(* Logix 5000 AddOnInstructionDefinition export Banner_TL70Pro_Param_v4; software revision 33.00; part 3 of 3 *)
(* tags used below, declared in another part *)
   TL70Pro : Banner_TL70Pro_v4;
   Port_Data : Banner_IOL_Port_v4;
   Port : INT;   // Port Number that device is plugged into.
   Local_Control : DINT;
   Command_Being_Processed : BOOL;
   Update_Archive : BOOL;
   Index_Write_Inprocess : DINT;
   Inprocess_Index : DINT;
   W_Index : DINT;
(* Banner_TL70Pro_Param_v4, continued *)

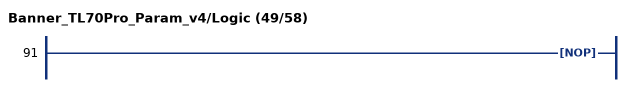
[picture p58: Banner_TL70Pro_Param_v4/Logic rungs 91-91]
   91: NOP();
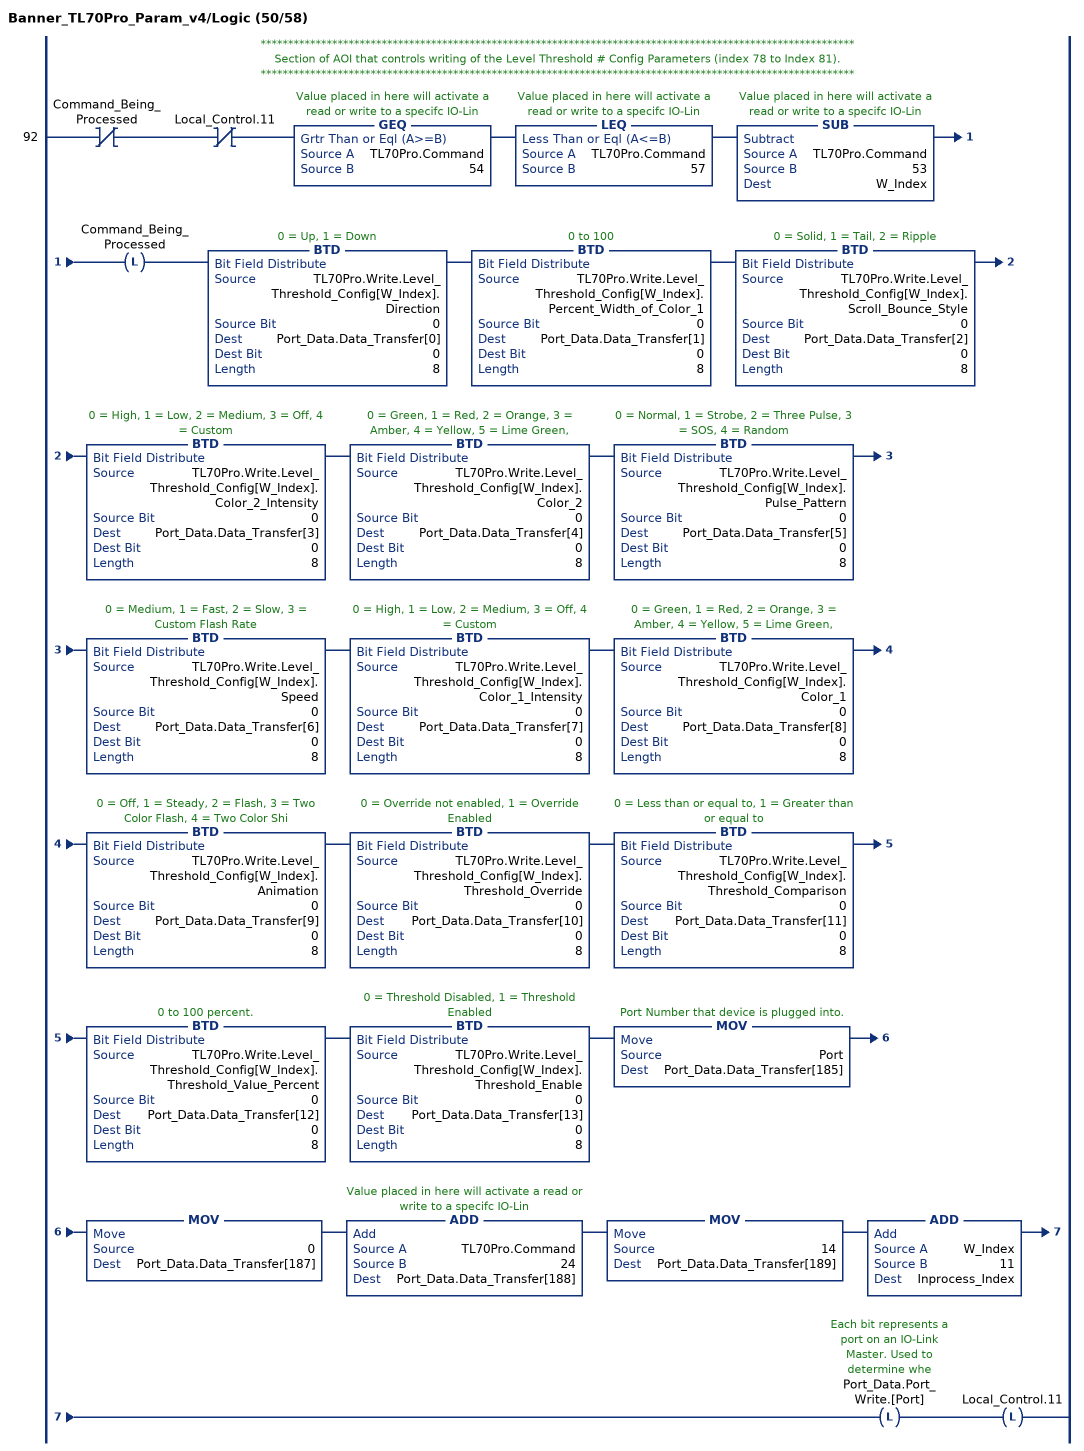
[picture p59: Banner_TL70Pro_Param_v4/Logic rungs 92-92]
   // ************************************************************************************************************
   // Section of AOI that controls writing of the Level Threshold # Config Parameters (index 78 to Index 81).
   // ************************************************************************************************************
   92: XIO(Command_Being_Processed)XIO(Local_Control.11)GEQ(TL70Pro.Command,54)LEQ(TL70Pro.Command,57)SUB(TL70Pro.Command,53,W_Index)OTL(Command_Being_Processed)BTD(TL70Pro.Write.Level_Threshold_Config[W_Index].Direction,0,Port_Data.Data_Transfer[0],0,8)BTD(TL70Pro.Write.Level_Threshold_Config[W_Index].Percent_Width_of_Color_1,0,Port_Data.Data_Transfer[1],0,8)BTD(TL70Pro.Write.Level_Threshold_Config[W_Index].Scroll_Bounce_Style,0,Port_Data.Data_Transfer[2],0,8)BTD(TL70Pro.Write.Level_Threshold_Config[W_Index].Color_2_Intensity,0,Port_Data.Data_Transfer[3],0,8)BTD(TL70Pro.Write.Level_Threshold_Config[W_Index].Color_2,0,Port_Data.Data_Transfer[4],0,8)BTD(TL70Pro.Write.Level_Threshold_Config[W_Index].Pulse_Pattern,0,Port_Data.Data_Transfer[5],0,8)BTD(TL70Pro.Write.Level_Threshold_Config[W_Index].Speed,0,Port_Data.Data_Transfer[6],0,8)BTD(TL70Pro.Write.Level_Threshold_Config[W_Index].Color_1_Intensity,0,Port_Data.Data_Transfer[7],0,8)BTD(TL70Pro.Write.Level_Threshold_Config[W_Index].Color_1,0,Port_Data.Data_Transfer[8],0,8)BTD(TL70Pro.Write.Level_Threshold_Config[W_Index].Animation,0,Port_Data.Data_Transfer[9],0,8)BTD(TL70Pro.Write.Level_Threshold_Config[W_Index].Threshold_Override,0,Port_Data.Data_Transfer[10],0,8)BTD(TL70Pro.Write.Level_Threshold_Config[W_Index].Threshold_Comparison,0,Port_Data.Data_Transfer[11],0,8)BTD(TL70Pro.Write.Level_Threshold_Config[W_Index].Threshold_Value_Percent,0,Port_Data.Data_Transfer[12],0,8)BTD(TL70Pro.Write.Level_Threshold_Config[W_Index].Threshold_Enable,0,Port_Data.Data_Transfer[13],0,8)MOV(Port,Port_Data.Data_Transfer[185])MOV(0,Port_Data.Data_Transfer[187])ADD(TL70Pro.Command,24,Port_Data.Data_Transfer[188])MOV(14,Port_Data.Data_Transfer[189])ADD(W_Index,11,Inprocess_Index)OTL(Port_Data.Port_Write.[Port])OTL(Local_Control.11);
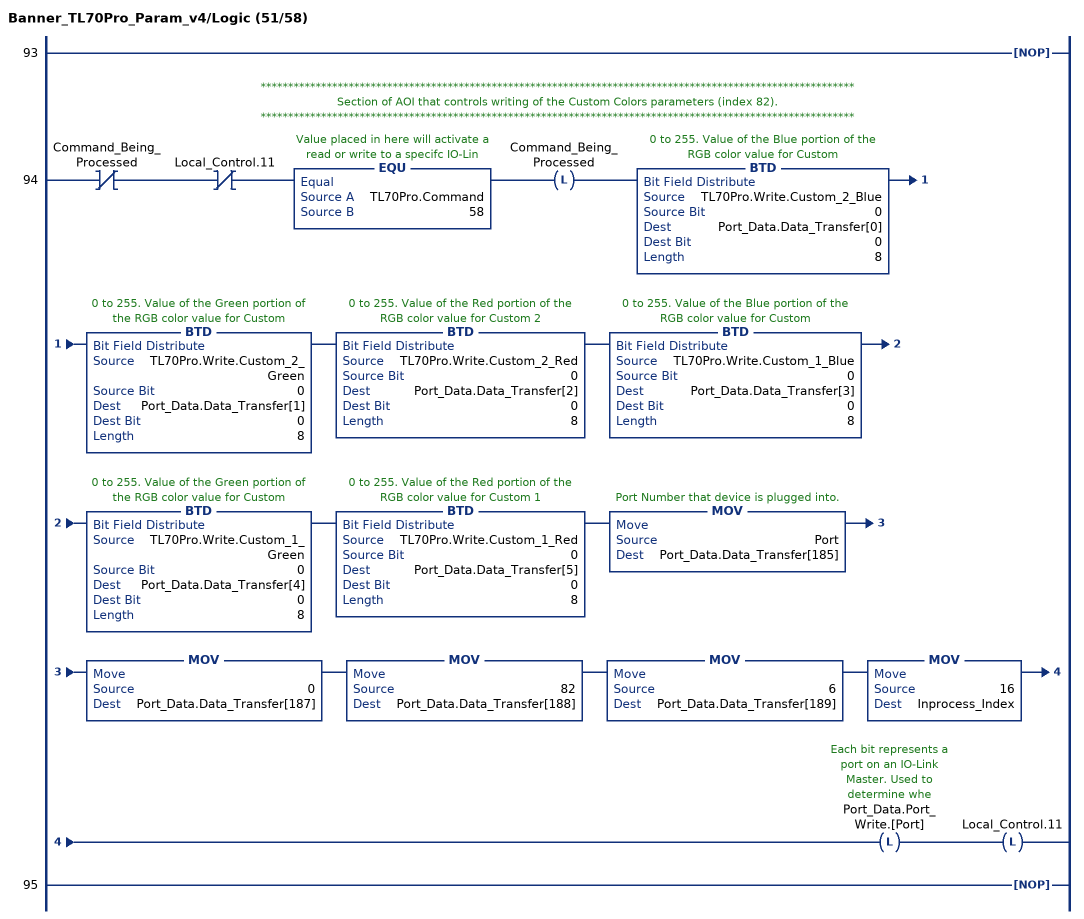
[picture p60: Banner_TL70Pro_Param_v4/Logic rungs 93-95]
   93: NOP();
   // ************************************************************************************************************
   // Section of AOI that controls writing of the Custom Colors parameters (index 82).
   // ************************************************************************************************************
   94: XIO(Command_Being_Processed)XIO(Local_Control.11)EQU(TL70Pro.Command,58)OTL(Command_Being_Processed)BTD(TL70Pro.Write.Custom_2_Blue,0,Port_Data.Data_Transfer[0],0,8)BTD(TL70Pro.Write.Custom_2_Green,0,Port_Data.Data_Transfer[1],0,8)BTD(TL70Pro.Write.Custom_2_Red,0,Port_Data.Data_Transfer[2],0,8)BTD(TL70Pro.Write.Custom_1_Blue,0,Port_Data.Data_Transfer[3],0,8)BTD(TL70Pro.Write.Custom_1_Green,0,Port_Data.Data_Transfer[4],0,8)BTD(TL70Pro.Write.Custom_1_Red,0,Port_Data.Data_Transfer[5],0,8)MOV(Port,Port_Data.Data_Transfer[185])MOV(0,Port_Data.Data_Transfer[187])MOV(82,Port_Data.Data_Transfer[188])MOV(6,Port_Data.Data_Transfer[189])MOV(16,Inprocess_Index)OTL(Port_Data.Port_Write.[Port])OTL(Local_Control.11);
   95: NOP();
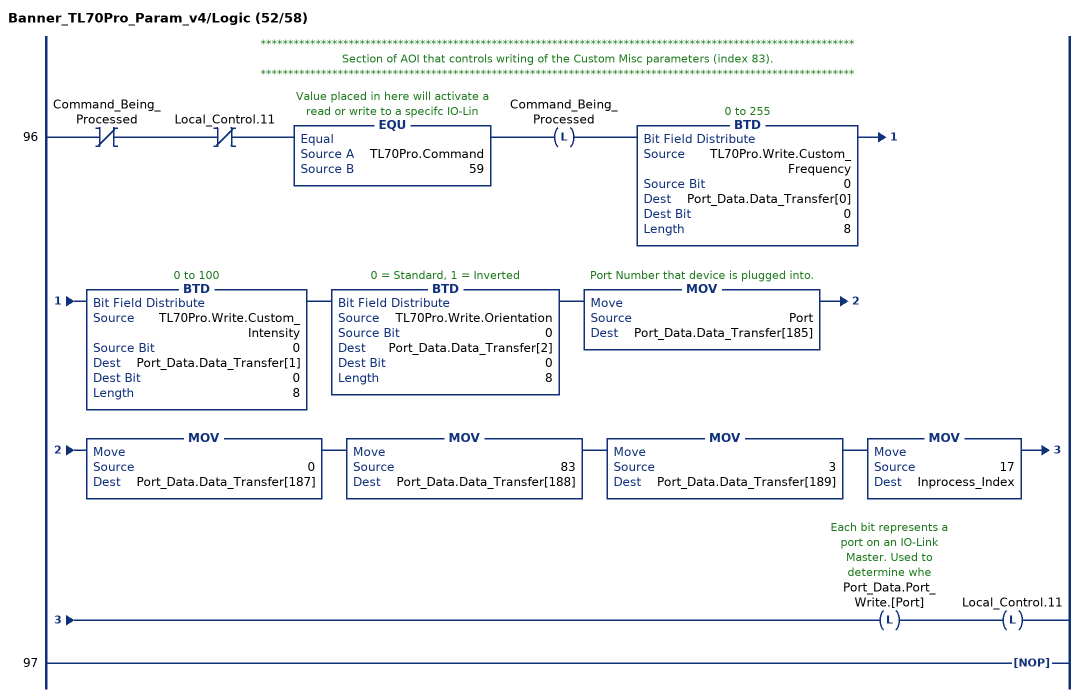
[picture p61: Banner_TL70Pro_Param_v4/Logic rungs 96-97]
   // ************************************************************************************************************
   // Section of AOI that controls writing of the Custom Misc parameters (index 83).
   // ************************************************************************************************************
   96: XIO(Command_Being_Processed)XIO(Local_Control.11)EQU(TL70Pro.Command,59)OTL(Command_Being_Processed)BTD(TL70Pro.Write.Custom_Frequency,0,Port_Data.Data_Transfer[0],0,8)BTD(TL70Pro.Write.Custom_Intensity,0,Port_Data.Data_Transfer[1],0,8)BTD(TL70Pro.Write.Orientation,0,Port_Data.Data_Transfer[2],0,8)MOV(Port,Port_Data.Data_Transfer[185])MOV(0,Port_Data.Data_Transfer[187])MOV(83,Port_Data.Data_Transfer[188])MOV(3,Port_Data.Data_Transfer[189])MOV(17,Inprocess_Index)OTL(Port_Data.Port_Write.[Port])OTL(Local_Control.11);
   97: NOP();
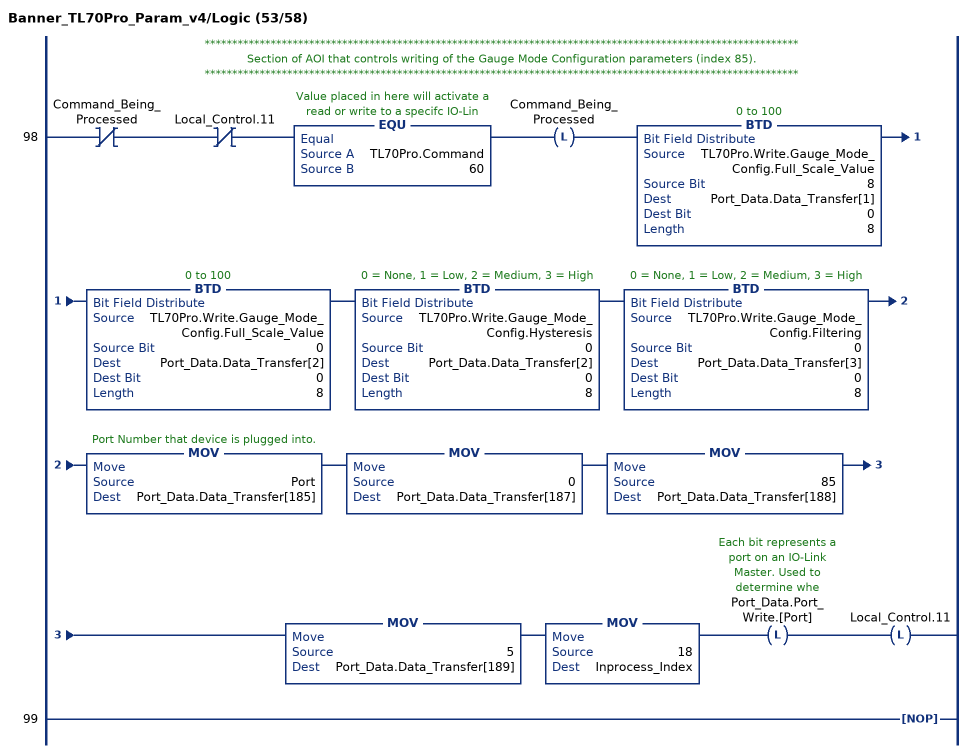
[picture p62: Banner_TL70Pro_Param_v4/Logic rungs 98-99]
   // ************************************************************************************************************
   // Section of AOI that controls writing of the Gauge Mode Configuration parameters (index 85).
   // ************************************************************************************************************
   98: XIO(Command_Being_Processed)XIO(Local_Control.11)EQU(TL70Pro.Command,60)OTL(Command_Being_Processed)BTD(TL70Pro.Write.Gauge_Mode_Config.Full_Scale_Value,8,Port_Data.Data_Transfer[1],0,8)BTD(TL70Pro.Write.Gauge_Mode_Config.Full_Scale_Value,0,Port_Data.Data_Transfer[2],0,8)BTD(TL70Pro.Write.Gauge_Mode_Config.Hysteresis,0,Port_Data.Data_Transfer[2],0,8)BTD(TL70Pro.Write.Gauge_Mode_Config.Filtering,0,Port_Data.Data_Transfer[3],0,8)MOV(Port,Port_Data.Data_Transfer[185])MOV(0,Port_Data.Data_Transfer[187])MOV(85,Port_Data.Data_Transfer[188])MOV(5,Port_Data.Data_Transfer[189])MOV(18,Inprocess_Index)OTL(Port_Data.Port_Write.[Port])OTL(Local_Control.11);
   99: NOP();
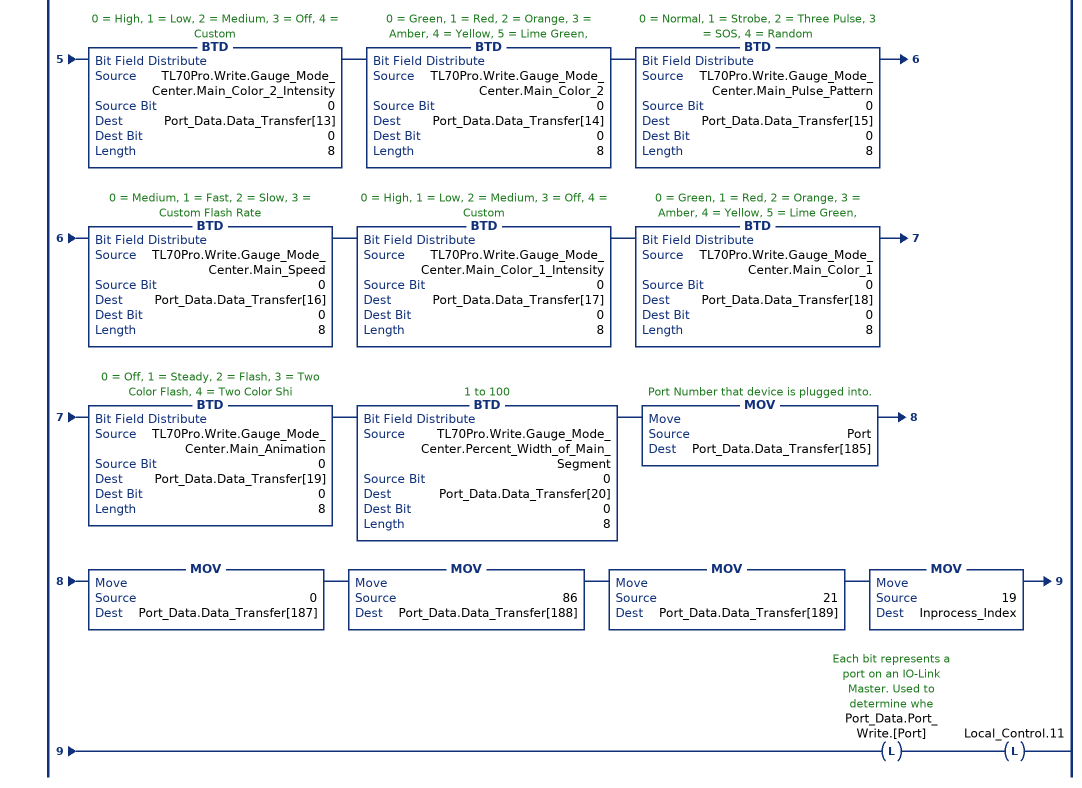
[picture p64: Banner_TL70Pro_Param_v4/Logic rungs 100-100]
   // ************************************************************************************************************
   // Section of AOI that controls writing of the Gauge Mode Center Settings parameters (index 86).
   // ************************************************************************************************************
   100: XIO(Command_Being_Processed)XIO(Local_Control.11)EQU(TL70Pro.Command,61)OTL(Command_Being_Processed)BTD(TL70Pro.Write.Gauge_Mode_Center.BG_Direction,0,Port_Data.Data_Transfer[0],0,8)BTD(TL70Pro.Write.Gauge_Mode_Center.BG_Percent_Width_of_Color_1,0,Port_Data.Data_Transfer[1],0,8)BTD(TL70Pro.Write.Gauge_Mode_Center.BG_Scroll_Bounce_Style,0,Port_Data.Data_Transfer[2],0,8)BTD(TL70Pro.Write.Gauge_Mode_Center.BG_Color_2_Intensity,0,Port_Data.Data_Transfer[3],0,8)BTD(TL70Pro.Write.Gauge_Mode_Center.BG_Color_2,0,Port_Data.Data_Transfer[4],0,8)BTD(TL70Pro.Write.Gauge_Mode_Center.BG_Pulse_Pattern,0,Port_Data.Data_Transfer[5],0,8)BTD(TL70Pro.Write.Gauge_Mode_Center.BG_Speed,0,Port_Data.Data_Transfer[6],0,8)BTD(TL70Pro.Write.Gauge_Mode_Center.BG_Color_1_Intensity,0,Port_Data.Data_Transfer[7],0,8)BTD(TL70Pro.Write.Gauge_Mode_Center.BG_Color_1,0,Port_Data.Data_Transfer[8],0,8)BTD(TL70Pro.Write.Gauge_Mode_Center.BG_Animation,0,Port_Data.Data_Transfer[9],0,8)BTD(TL70Pro.Write.Gauge_Mode_Center.Main_Direction,0,Port_Data.Data_Transfer[10],0,8)BTD(TL70Pro.Write.Gauge_Mode_Center.Main_Percent_Width_of_Color_1,0,Port_Data.Data_Transfer[11],0,8)BTD(TL70Pro.Write.Gauge_Mode_Center.Main_Scroll_Bounce_Style,0,Port_Data.Data_Transfer[12],0,8)BTD(TL70Pro.Write.Gauge_Mode_Center.Main_Color_2_Intensity,0,Port_Data.Data_Transfer[13],0,8)BTD(TL70Pro.Write.Gauge_Mode_Center.Main_Color_2,0,Port_Data.Data_Transfer[14],0,8)BTD(TL70Pro.Write.Gauge_Mode_Center.Main_Pulse_Pattern,0,Port_Data.Data_Transfer[15],0,8)BTD(TL70Pro.Write.Gauge_Mode_Center.Main_Speed,0,Port_Data.Data_Transfer[16],0,8)BTD(TL70Pro.Write.Gauge_Mode_Center.Main_Color_1_Intensity,0,Port_Data.Data_Transfer[17],0,8)BTD(TL70Pro.Write.Gauge_Mode_Center.Main_Color_1,0,Port_Data.Data_Transfer[18],0,8)BTD(TL70Pro.Write.Gauge_Mode_Center.Main_Animation,0,Port_Data.Data_Transfer[19],0,8)BTD(TL70Pro.Write.Gauge_Mode_Center.Percent_Width_of_Main_Segment,0,Port_Data.Data_Transfer[20],0,8)MOV(Port,Port_Data.Data_Transfer[185])MOV(0,Port_Data.Data_Transfer[187])MOV(86,Port_Data.Data_Transfer[188])MOV(21,Port_Data.Data_Transfer[189])MOV(19,Inprocess_Index)OTL(Port_Data.Port_Write.[Port])OTL(Local_Control.11);
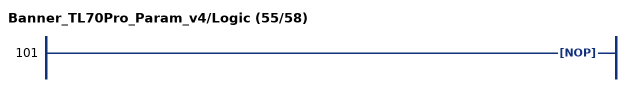
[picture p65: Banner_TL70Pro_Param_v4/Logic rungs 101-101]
   101: NOP();
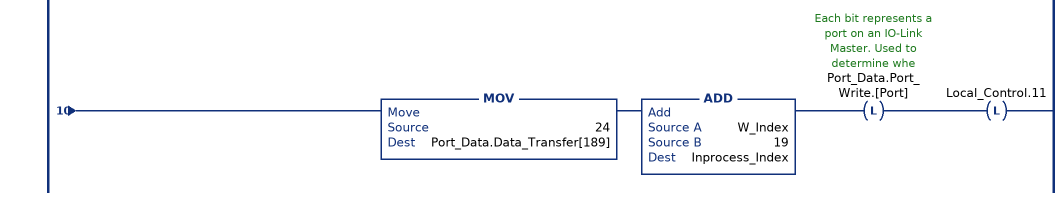
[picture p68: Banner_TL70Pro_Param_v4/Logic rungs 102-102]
   // ************************************************************************************************************
   // Section of AOI that controls writing of the Gauge Mode Threshold # Settings Parameters (index 87 to Index 88).
   // ************************************************************************************************************
   102: XIO(Command_Being_Processed)XIO(Local_Control.11)GEQ(TL70Pro.Command,62)LEQ(TL70Pro.Command,63)SUB(TL70Pro.Command,61,W_Index)OTL(Command_Being_Processed)BTD(TL70Pro.Write.Gauge_Mode_Threshold[W_Index].BG_Direction,0,Port_Data.Data_Transfer[0],0,8)BTD(TL70Pro.Write.Gauge_Mode_Threshold[W_Index].BG_Percent_Width_of_Color_1,0,Port_Data.Data_Transfer[1],0,8)BTD(TL70Pro.Write.Gauge_Mode_Threshold[W_Index].BG_Scroll_Bounce_Style,0,Port_Data.Data_Transfer[2],0,8)BTD(TL70Pro.Write.Gauge_Mode_Threshold[W_Index].BG_Color_2_Intensity,0,Port_Data.Data_Transfer[3],0,8)BTD(TL70Pro.Write.Gauge_Mode_Threshold[W_Index].BG_Color_2,0,Port_Data.Data_Transfer[4],0,8)BTD(TL70Pro.Write.Gauge_Mode_Threshold[W_Index].BG_Pulse_Pattern,0,Port_Data.Data_Transfer[5],0,8)BTD(TL70Pro.Write.Gauge_Mode_Threshold[W_Index].BG_Speed,0,Port_Data.Data_Transfer[6],0,8)BTD(TL70Pro.Write.Gauge_Mode_Threshold[W_Index].BG_Color_1_Intensity,0,Port_Data.Data_Transfer[7],0,8)BTD(TL70Pro.Write.Gauge_Mode_Threshold[W_Index].BG_Color_1,0,Port_Data.Data_Transfer[8],0,8)BTD(TL70Pro.Write.Gauge_Mode_Threshold[W_Index].BG_Animation,0,Port_Data.Data_Transfer[9],0,8)BTD(TL70Pro.Write.Gauge_Mode_Threshold[W_Index].Main_Direction,0,Port_Data.Data_Transfer[10],0,8)BTD(TL70Pro.Write.Gauge_Mode_Threshold[W_Index].Main_Percent_Width_of_Color_1,0,Port_Data.Data_Transfer[11],0,8)BTD(TL70Pro.Write.Gauge_Mode_Threshold[W_Index].Main_Scroll_Bounce_Style,0,Port_Data.Data_Transfer[12],0,8)BTD(TL70Pro.Write.Gauge_Mode_Threshold[W_Index].Main_Color_2_Intensity,0,Port_Data.Data_Transfer[13],0,8)BTD(TL70Pro.Write.Gauge_Mode_Threshold[W_Index].Main_Color_2,0,Port_Data.Data_Transfer[14],0,8)BTD(TL70Pro.Write.Gauge_Mode_Threshold[W_Index].Main_Pulse_Pattern,0,Port_Data.Data_Transfer[15],0,8)BTD(TL70Pro.Write.Gauge_Mode_Threshold[W_Index].Main_Speed,0,Port_Data.Data_Transfer[16],0,8)BTD(TL70Pro.Write.Gauge_Mode_Threshold[W_Index].Main_Color_1_Intensity,0,Port_Data.Data_Transfer[17],0,8)BTD(TL70Pro.Write.Gauge_Mode_Threshold[W_Index].Main_Color_1,0,Port_Data.Data_Transfer[18],0,8)BTD(TL70Pro.Write.Gauge_Mode_Threshold[W_Index].Main_Animation,0,Port_Data.Data_Transfer[19],0,8)BTD(TL70Pro.Write.Gauge_Mode_Threshold[W_Index].Percent_Width_of_Main_Segment,0,Port_Data.Data_Transfer[20],0,8)BTD(TL70Pro.Write.Gauge_Mode_Threshold[W_Index].Threshold_Comparison,0,Port_Data.Data_Transfer[21],0,8)BTD(TL70Pro.Write.Gauge_Mode_Threshold[W_Index].Threshold_Value,0,Port_Data.Data_Transfer[22],0,8)BTD(TL70Pro.Write.Gauge_Mode_Threshold[W_Index].Threshold_Enable,0,Port_Data.Data_Transfer[23],0,8)MOV(Port,Port_Data.Data_Transfer[185])MOV(0,Port_Data.Data_Transfer[187])ADD(TL70Pro.Command,25,Port_Data.Data_Transfer[188])MOV(24,Port_Data.Data_Transfer[189])ADD(W_Index,19,Inprocess_Index)OTL(Port_Data.Port_Write.[Port])OTL(Local_Control.11);
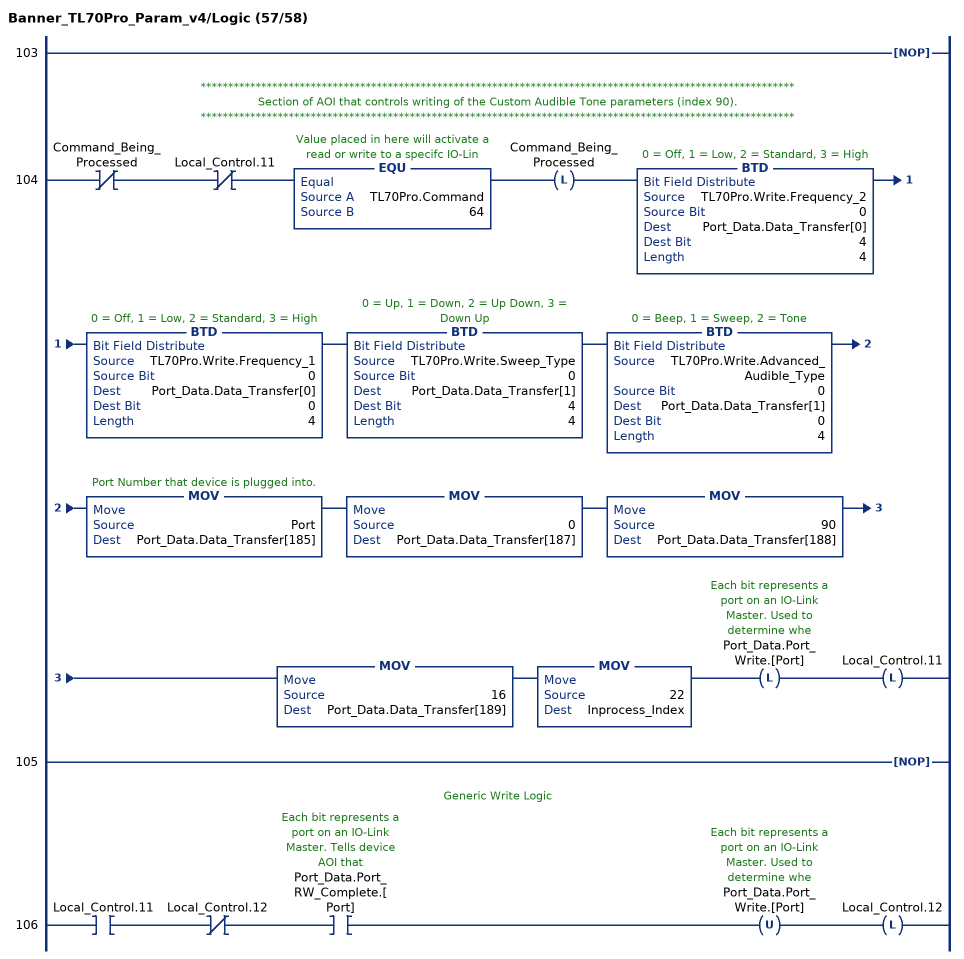
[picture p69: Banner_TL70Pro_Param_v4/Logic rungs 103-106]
   103: NOP();
   // ************************************************************************************************************
   // Section of AOI that controls writing of the Custom Audible Tone parameters (index 90).
   // ************************************************************************************************************
   104: XIO(Command_Being_Processed)XIO(Local_Control.11)EQU(TL70Pro.Command,64)OTL(Command_Being_Processed)BTD(TL70Pro.Write.Frequency_2,0,Port_Data.Data_Transfer[0],4,4)BTD(TL70Pro.Write.Frequency_1,0,Port_Data.Data_Transfer[0],0,4)BTD(TL70Pro.Write.Sweep_Type,0,Port_Data.Data_Transfer[1],4,4)BTD(TL70Pro.Write.Advanced_Audible_Type,0,Port_Data.Data_Transfer[1],0,4)MOV(Port,Port_Data.Data_Transfer[185])MOV(0,Port_Data.Data_Transfer[187])MOV(90,Port_Data.Data_Transfer[188])MOV(16,Port_Data.Data_Transfer[189])MOV(22,Inprocess_Index)OTL(Port_Data.Port_Write.[Port])OTL(Local_Control.11);
   105: NOP();
   // Generic Write Logic
   106: XIC(Local_Control.11)XIO(Local_Control.12)XIC(Port_Data.Port_RW_Complete.[Port])OTU(Port_Data.Port_Write.[Port])OTL(Local_Control.12);
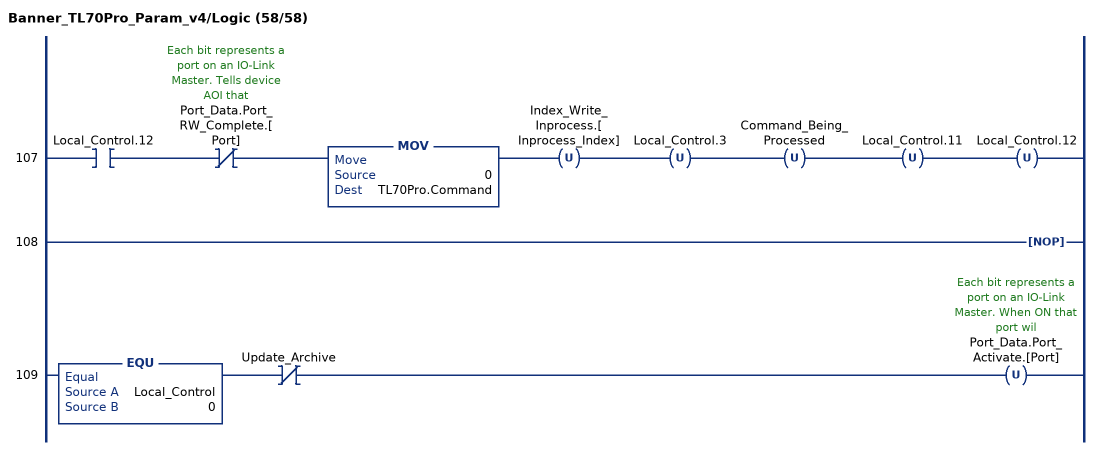
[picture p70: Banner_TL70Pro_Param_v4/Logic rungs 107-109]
   107: XIC(Local_Control.12)XIO(Port_Data.Port_RW_Complete.[Port])MOV(0,TL70Pro.Command)OTU(Index_Write_Inprocess.[Inprocess_Index])OTU(Local_Control.3)OTU(Command_Being_Processed)OTU(Local_Control.11)OTU(Local_Control.12);
   108: NOP();
   109: EQU(Local_Control,0)XIO(Update_Archive)OTU(Port_Data.Port_Activate.[Port]);
END_ROUTINE
END_ADD_ON_INSTRUCTION
